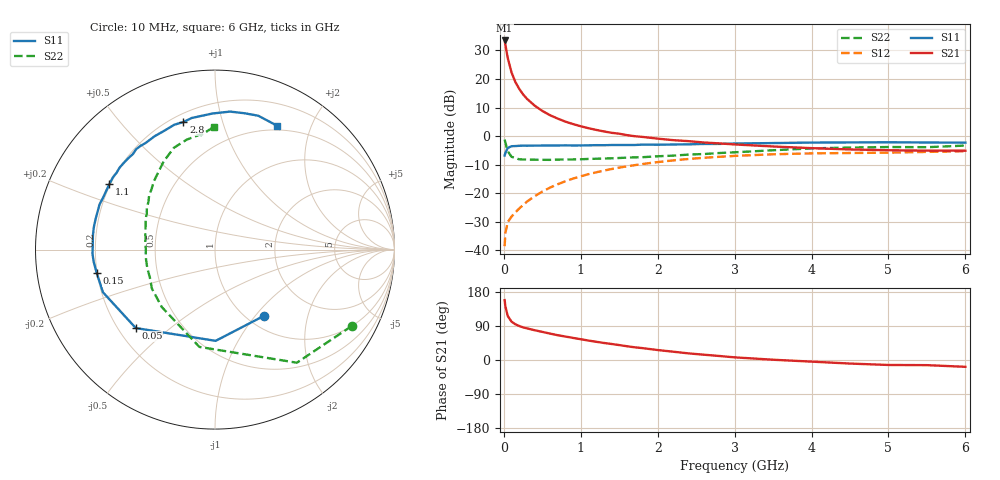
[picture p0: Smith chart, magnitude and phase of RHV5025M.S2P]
! SIEMENS Small Signal Semiconductors
! BFR106
! Si NPN RF Bipolar Junction Transistor in SOT23
! VCE = 0.5 V  IC = 25 mA
! Common Emitter S-Parameters:  August  1996
# GHz  S  MA  R  50
!  f  S11  S21  S12  S22
! GHz  MAG  ANG  MAG  ANG  MAG  ANG  MAG  ANG
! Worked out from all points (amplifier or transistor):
!   36 points, 10 MHz to 6 GHz, reference 50 ohm
!   highest |S21| = 33.5 dB at 10 MHz (marker M1)
!   |S21| within 3 dB of that: start of sweep to 30.04 MHz
!   unconditionally stable (mu >= 1): 261.8 MHz to end of sweep
!   at 250 MHz: K = 0.99, MSG = 19.4 dB, |S12| = -24.1 dB
!   at 1.4 GHz: K = 1.10, MAG = 4.4 dB, |S12| = -11.5 dB
!   at 6 GHz: K = 1.03, MAG = -1.0 dB, |S12| = -5.3 dB
!   S11 on the Smith chart (normalised r, x): 10 MHz: 1.19, -1.11; 50 MHz: 0.27, -0.39; 150 MHz: 0.20, -0.09; 1.1 GHz: 0.20, +0.27; 2.8 GHz: 0.25, +0.75; 6 GHz: 0.45, +1.53
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0.01  0.4588 -53.6  47.35 158.1  0.0119 72.3  0.8727 -29.2
0.02  0.5085 -89.6  40.03 141.8  0.0201 60.3  0.7781 -54.1
0.05  0.6212 -135.3  23.56 116.3  0.0312 45.2  0.5491 -99.1
0.1  0.6679 -159.1  13.05 101.2  0.0392 44.9  0.4362 -132.8
0.15  0.6719 -168.8  8.863 94.2  0.0465 48.3  0.4132 -148.4
0.2  0.6793 -174.2  6.734 89.7  0.0543 52.6  0.3945 -157.0
0.25  0.6829 -178.1  5.39 86.1  0.0623 56.0  0.3913 -163.3
0.3  0.6814 178.9  4.514 83.5  0.0715 58.0  0.3896 -167.2
0.4  0.6847 173.4  3.43 78.6  0.0891 60.8  0.388 -173.4
0.5  0.6866 169.6  2.77 74.2  0.1072 61.9  0.386 -177.8
0.6  0.6867 165.2  2.332 69.7  0.126 61.8  0.3854 179.0
0.7  0.6877 161.6  2.032 65.4  0.1443 61.4  0.3894 176.3
0.9  0.6875 155.0  1.629 58.3  0.1813 59.2  0.3919 170.7
1.1  0.6925 148.3  1.381 51.3  0.2163 56.6  0.4 166.8
1.3  0.6957 142.0  1.212 45.0  0.25 53.1  0.4064 162.2
1.6  0.7019 133.6  1.044 36.3  0.2969 48.0  0.4212 156.3
2.2  0.7157 118.0  0.853 21.9  0.3771 37.2  0.4567 144.3
2.8  0.7323 103.9  0.748 10.6  0.4357 26.7  0.5077 132.5
3.5  0.7583 91.1  0.661 0.7  0.4826 15.7  0.5677 120.3
4.5  0.7774 77.7  0.586 -9.4  0.5082 2.4  0.6324 104.5
5.5  0.7753 67.4  0.559 -13.6  0.5311 -5.5  0.6422 96.9
6  0.772 63.4  0.558 -18.0  0.5452 -11.6  0.6852 90.4
